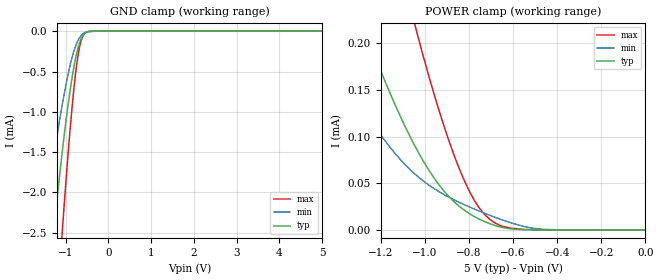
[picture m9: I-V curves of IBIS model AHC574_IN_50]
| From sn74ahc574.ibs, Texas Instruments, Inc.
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[Model]   AHC574_IN_50
Model_type  Input
Vinl = 1.65
Vinh = 3.85
| variable   typ   min   max
C_comp   1.34pF   0.87pF   1.62pF
[Temperature Range]   40   100   -40
| Ambient temperature   25   85   -40
[Voltage range]   5   4.5   5.5
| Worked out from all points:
|   GND clamp passes 1 mA (typ) near -0.97 V on its own axis
|   POWER clamp passes 1 mA (typ) near -2.22 V on its own axis
[GND Clamp]
| AHC574_IN_50
|   Voltage   I(typ)   I(min)   I(max)
-5V       -31.77mA   -20.73mA   -40.38mA
-1.565V   -4.109mA   -2.618mA   -6.471mA
-1.515V   -3.807mA   -2.422mA   -6.033mA
-1.285V   -2.505mA   -1.573mA   -4.084mA
-1.085V   -1.512mA   -922.5uA   -2.513mA
-1.065V   -1.421mA   -863.1uA   -2.364mA
-905mV    -763.5uA   -439.9uA   -1.264mA
-775mV    -351.6uA   -192.7uA   -547.4uA
-675mV    -141.8uA   -79.64uA   -193.1uA
-625mV    -77.12uA   -46.27uA   -95.01uA
-555mV    -27.17uA   -18.51uA   -28.04uA
5V        10.5nA     1.523uA    97.28nA
[POWER Clamp]
| AHC574_IN_50
|   Voltage   I(typ)   I(min)   I(max)
-5V       4.331mA    2.882mA    6.871mA
-1.495V   368.8uA    224.2uA    713.6uA
-1.46V    343.2uA    207.8uA    670.4uA
-1.28V    220.2uA    131uA      459.5uA
-1.055V   94.9uA     62.27uA    229.6uA
-1.03V    83.76uA    57.04uA    207uA
-935mV    48.36uA    41.06uA    128.2uA
-850mV    26.7uA     30.4uA     69.72uA
-775mV    14.38uA    22.45uA    31.74uA
-705mV    6.746uA    15.74uA    11.35uA
-465mV    30.11nA    671.2nA    253.5nA
-84.45fV  10.5nA     614.6pA    148.7nA
